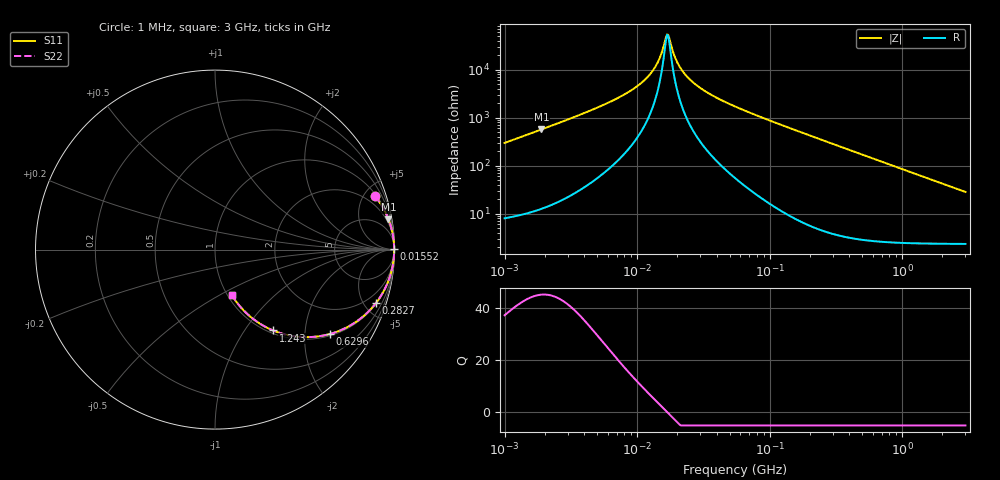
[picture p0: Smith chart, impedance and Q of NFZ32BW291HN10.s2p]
! NFZ32BW291HN10
# Hz S RI R 50
!Freq.(Hz) S11(Real) S11(Imag) S21(Real) S21(Imag) S12(Real) S12(Imag) S22(Real) S22(Imag)
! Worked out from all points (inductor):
!   401 points, 1 MHz to 3 GHz, reference 50 ohm
!   read as one part in series: L = 47 uH near 1.041 MHz
!   highest Q = 45 at 1.897 MHz (marker M1), where L = 47.6 uH
!   self-resonance near 16.81 MHz
!   S11 on the Smith chart (normalised r, x): 1 MHz: 1.16, +5.94; 15.52 MHz: open; 282.7 MHz: 1.08, -6.01; 629.6 MHz: 1.05, -2.69; 1.243 GHz: 1.05, -1.36; 3 GHz: 1.05, -0.56
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1000000  0.8919 0.2974  0.1081 -0.2974  0.1081 -0.2974  0.8919 0.2974
1897447  0.9663 0.1697  0.0337 -0.1697  0.0337 -0.1697  0.9663 0.1697
3823119  0.9907 0.0832  0.00931 -0.0832  0.00931 -0.0832  0.9907 0.0832
6696013  0.9962 0.0425  0.00377 -0.0425  0.00377 -0.0425  0.9962 0.0425
9600343  0.9976 0.0239  0.00245 -0.0239  0.00245 -0.0239  0.9976 0.0239
1.245355e7  0.998 0.0125  0.002 -0.0125  0.002 -0.0125  0.998 0.0125
1.461624e7  0.9981 0.00593  0.00186 -0.00593  0.00186 -0.00593  0.9981 0.00593
1.55208e7  0.9982 0.00352  0.00184 -0.00352  0.00184 -0.00352  0.9982 0.00352
1.648134e7  0.9982 0.00112  0.00182 -0.00112  0.00182 -0.00112  0.9982 0.00112
1.71545e7  0.9982 -0.000477  0.00182 0.000477  0.00182 0.000477  0.9982 -0.000477
2.013356e7  0.9981 -0.0069  0.00187 0.0069  0.00187 0.0069  0.9981 -0.0069
2.181181e7  0.9981 -0.0102  0.00192 0.0102  0.00192 0.0102  0.9981 -0.0102
2.459509e7  0.998 -0.0152  0.00205 0.0152  0.00205 0.0152  0.998 -0.0152
3.387922e7  0.9973 -0.0299  0.00272 0.0299  0.00272 0.0299  0.9973 -0.0299
5.477226e7  0.9947 -0.0581  0.00527 0.0581  0.00527 0.0581  0.9947 -0.0581
2.094008e8  0.9404 -0.2303  0.0596 0.2303  0.0596 0.2303  0.9404 -0.2303
2.827291e8  0.8972 -0.2971  0.1028 0.2971  0.1028 0.2971  0.8972 -0.2971
6.296259e8  0.6417 -0.4697  0.3583 0.4697  0.3583 0.4697  0.6417 -0.4697
8.005644e8  0.5278 -0.4874  0.4722 0.4874  0.4722 0.4874  0.5278 -0.4874
1.243477e9  0.323 -0.4503  0.677 0.4503  0.677 0.4503  0.323 -0.4503
1.893158e9  0.1797 -0.3585  0.8203 0.3585  0.8203 0.3585  0.1797 -0.3585
3e9  0.092 -0.2505  0.908 0.2505  0.908 0.2505  0.092 -0.2505
